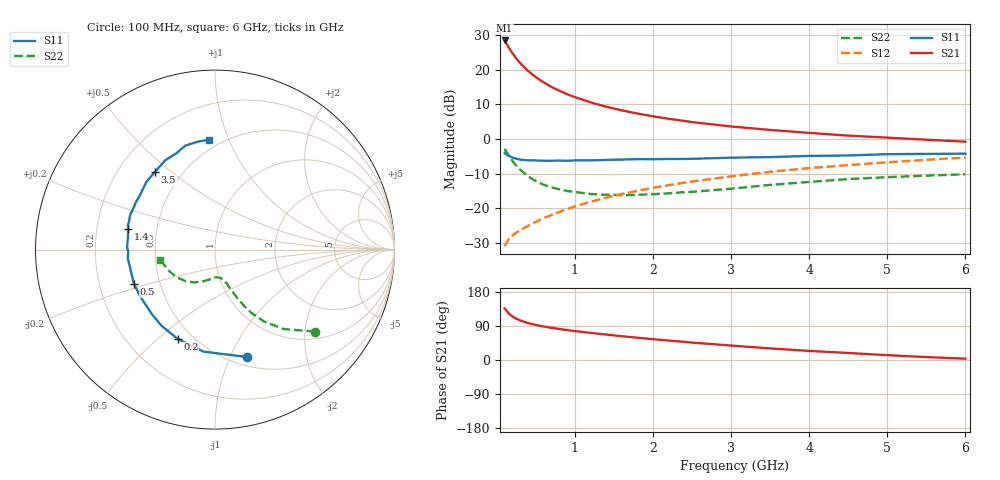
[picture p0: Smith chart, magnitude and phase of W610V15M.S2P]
! SIEMENS Small Signal Semiconductors
! BFR193W
! Si NPN RF Bipolar Junction Transistor in SOT323
! VCE = 10 V  IC = 15 mA
! Common Emitter S-Parameters:  September  1992
# GHz  S  MA  R  50
!  f  S11  S21  S12  S22
! GHz  MAG  ANG  MAG  ANG  MAG  ANG  MAG  ANG
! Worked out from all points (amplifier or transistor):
!   28 points, 100 MHz to 6 GHz, reference 50 ohm
!   highest |S21| = 28.4 dB at 100 MHz (marker M1)
!   |S21| within 3 dB of that: start of sweep to 180.7 MHz
!   unconditionally stable (mu >= 1): 881.9 MHz to 2.65 GHz
!   at 300 MHz: K = 0.66, MSG = 24.1 dB, |S12| = -26.3 dB
!   at 1.5 GHz: K = 1.04, MAG = 11.4 dB, |S12| = -16.4 dB
!   at 6 GHz: K = 0.90, MSG = 2.3 dB, |S12| = -5.4 dB
!   S11 on the Smith chart (normalised r, x): 100 MHz: 0.59, -1.16; 200 MHz: 0.42, -0.58; 500 MHz: 0.36, -0.18; 1.4 GHz: 0.34, +0.10; 3.5 GHz: 0.36, +0.44; 6 GHz: 0.43, +0.85
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0.1  0.6254 -73.2  26.34 136.0  0.0284 59.8  0.7213 -39.3
0.15  0.572 -96.4  21.08 123.5  0.0355 54.7  0.5834 -49.3
0.2  0.539 -112.8  17.26 114.9  0.0405 52.7  0.4845 -55.7
0.25  0.5182 -125.1  14.46 108.9  0.0447 52.5  0.4098 -59.9
0.3  0.503 -134.2  12.4 104.3  0.0484 53.4  0.3598 -62.4
0.4  0.4917 -148.0  9.561 97.5  0.0558 55.4  0.2889 -65.7
0.5  0.4898 -156.9  7.773 92.5  0.0637 57.5  0.2463 -67.6
0.6  0.4845 -163.9  6.544 88.5  0.072 59.6  0.2187 -69.7
0.7  0.484 -169.5  5.622 84.9  0.08 61.2  0.2004 -70.8
0.8  0.4887 -174.2  4.962 81.8  0.0885 62.2  0.1878 -72.6
0.9  0.4837 -178.4  4.422 79.0  0.0975 63.2  0.1773 -73.5
1  0.4901 178.2  4.014 76.3  0.1062 63.9  0.1717 -75.1
1.2  0.4902 171.5  3.373 71.6  0.1242 64.6  0.1608 -78.9
1.4  0.4979 166.7  2.919 67.2  0.1419 64.8  0.1568 -82.4
1.8  0.5108 157.8  2.326 58.8  0.1784 64.1  0.1562 -90.4
2.2  0.5139 149.2  1.952 51.3  0.2153 62.6  0.1642 -97.3
2.5  0.5171 143.7  1.75 46.0  0.243 61.1  0.1725 -102.7
3  0.5371 135.4  1.513 38.1  0.289 58.1  0.1916 -111.8
3.5  0.547 127.7  1.349 30.6  0.3359 54.5  0.2173 -122.8
4.5  0.5777 112.0  1.116 18.5  0.4192 46.6  0.2635 -144.2
5.5  0.609 99.0  0.974 7.7  0.5002 38.5  0.2953 -163.2
6  0.613 93.0  0.913 3.5  0.5392 34.0  0.3098 -169.3
